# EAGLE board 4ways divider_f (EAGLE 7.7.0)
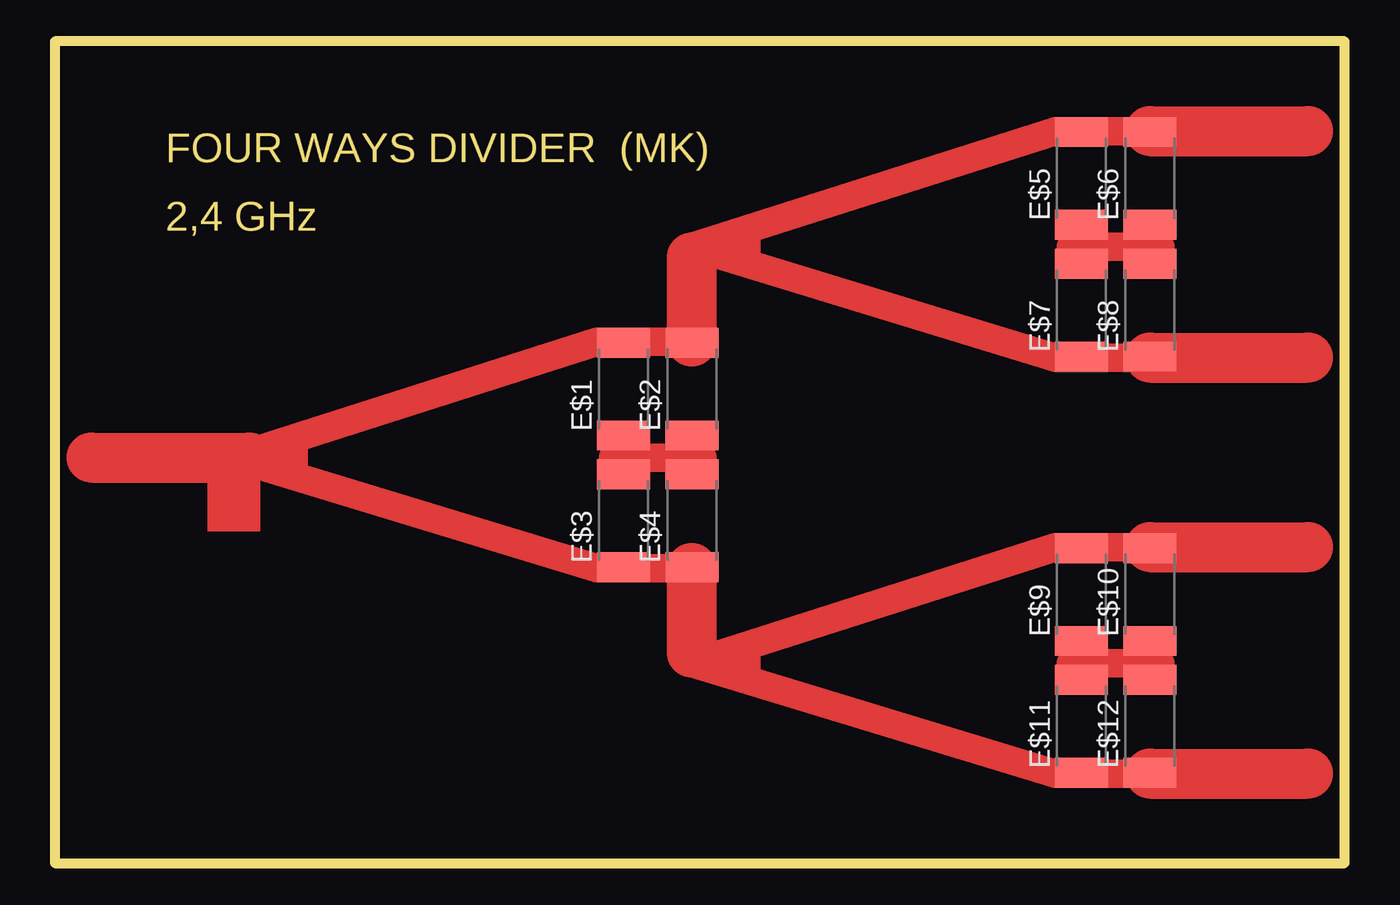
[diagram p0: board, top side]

Size 77.79 x 49.53 mm. Coordinates in mm from the lower left corner, seen from the top.
Outline: 0,0 77.79,0 77.79,49.53 0,49.53 0,0
Copper layers (1*16): Top 0.035mm / dielectric 1.5mm / Bottom 0.035mm
Design rules "default": minimum track width 10mil, minimum drill 24mil, track to track 8mil, track to pad 8mil, pad to pad 8mil, via to via 8mil, smd to smd 8mil, copper to edge 40mil, drill to drill 8mil, minimum pad ring 10mil, minimum via ring 8mil, stop-mask expansion 4mil, vias tented up to drill 0mil, thermal gap 10mil

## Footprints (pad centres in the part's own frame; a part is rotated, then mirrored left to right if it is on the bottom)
R2512 = smd 1.8 x 3.2: 1 -2.8,0; 2 2.8,0

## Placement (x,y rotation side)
E$1  [R2512]  34.29,28.57 90 top
E$2  [R2512]  38.42,28.57 90 top
E$3  [R2512]  34.29,20.64 90 top
E$4  [R2512]  38.42,20.64 90 top
E$5  [R2512]  61.91,41.27 90 top
E$6  [R2512]  66.04,41.27 90 top
E$7  [R2512]  61.91,33.34 90 top
E$8  [R2512]  66.04,33.34 90 top
E$9  [R2512]  61.91,16.19 90 top
E$10  [R2512]  66.04,16.19 90 top
E$11  [R2512]  61.91,8.26 90 top
E$12  [R2512]  66.04,8.26 90 top

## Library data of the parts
E$1-E$12 = rcl

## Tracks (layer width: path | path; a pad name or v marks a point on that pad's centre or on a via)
S$1
  Top 1.721: 32.7,31.43 10.79,24.45 32.7,17.78
S$2
  Top 1.721: 33.02,17.78 38.73,17.78
S$3
  Top 1.721: 33.66,24.45 39.05,24.45
S$4
  Top 1.721: 60.33,44.13 38.42,37.15 60.33,30.48
S$5
  Top 1.721: 60.64,30.48 66.36,30.48
S$6
  Top 1.721: 61.28,37.15 66.67,37.15
S$7
  Top 1.721: 33.34,31.43 38.42,31.43
  Top 3.024: 38.42,31.43 38.42,36.51
S$8
  Top 1.721: 60.96,44.13 66.04,44.13 66.67,44.13
  Top 3.024: 66.04,44.13 75.56,44.13 | 66.04,30.48 75.56,30.48 | 66.04,19.05 75.56,19.05 | 66.04,5.4 75.56,5.4 | 2.22,24.45 11.75,24.45
S$9
  Top 1.721: 60.33,19.05 38.42,12.06 60.33,5.4
S$10
  Top 1.721: 60.64,5.4 66.36,5.4
S$11
  Top 1.721: 61.28,12.06 66.67,12.06
S$12
  Top 1.721: 60.96,19.05 66.67,19.05
S$13
  Top 3.024: 38.42,12.7 38.42,17.78
(copper drawn outside any net)
  shapes: Top area x4

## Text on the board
Dimension: FOUR WAYS DIVIDER (MK) | 2,4 GHz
